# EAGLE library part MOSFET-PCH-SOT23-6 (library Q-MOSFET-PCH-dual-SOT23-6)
Dual P channel MOSFETs in an SOT23-6
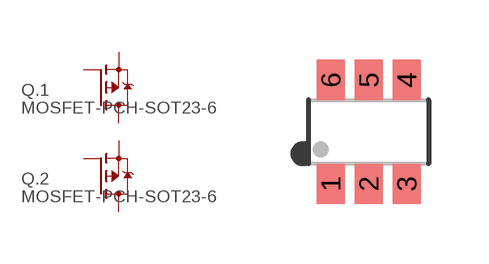
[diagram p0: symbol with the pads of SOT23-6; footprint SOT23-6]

Designator prefix Q; gates .1=P-MOSFET .2=P-MOSFET

## MOSFET-PCH-SOT23-6  [SOT23-6]
1  .1:G  pas
2  .2:S  pas
3  .2:G  pas
4  .2:D  pas
5  .1:S  pas
6  .1:D  pas

## Footprint SOT23-6 (pad centres in mm)
SOT23-6 Small Outline Transistor, standard 6-pin package
smd 0.7 x 1: 1 -0.95,-1.3; 2 0,-1.3; 3 0.95,-1.3; 4 0.95,1.3; 5 0,1.3; 6 -0.95,1.3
